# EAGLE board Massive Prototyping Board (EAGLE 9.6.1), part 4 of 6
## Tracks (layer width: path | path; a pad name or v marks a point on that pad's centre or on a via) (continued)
N$1187  (via drill 0.94) (continued)
  Bottom 2.032: v201.93,172.72 v204.47,172.72 v207.01,172.72 v209.55,172.72 v212.09,172.72
N$1188  (via drill 0.94)
  Bottom 2.032: v201.93,175.26 v204.47,175.26 v207.01,175.26 v209.55,175.26 v212.09,175.26
N$1189  (via drill 0.94)
  Bottom 2.032: v201.93,177.8 v204.47,177.8 v207.01,177.8 v209.55,177.8 v212.09,177.8
N$1190  (via drill 0.94)
  Bottom 2.032: v201.93,180.34 v204.47,180.34 v207.01,180.34 v209.55,180.34 v212.09,180.34
N$1191  (via drill 0.94)
  Bottom 2.032: v201.93,182.88 v204.47,182.88 v207.01,182.88 v209.55,182.88 v212.09,182.88
N$1192  (via drill 0.94)
  Bottom 2.032: v201.93,185.42 v204.47,185.42 v207.01,185.42 v209.55,185.42 v212.09,185.42
N$1193  (via drill 0.94)
  Bottom 2.032: v201.93,187.96 v204.47,187.96 v207.01,187.96 v209.55,187.96 v212.09,187.96
N$1194  (via drill 0.94)
  Bottom 2.032: v201.93,190.5 v204.47,190.5 v207.01,190.5 v209.55,190.5 v212.09,190.5
N$1195  (via drill 0.94)
  Bottom 2.032: v201.93,193.04 v204.47,193.04 v207.01,193.04 v209.55,193.04 v212.09,193.04
N$1196  (via drill 0.94)
  Bottom 2.032: v201.93,195.58 v204.47,195.58 v207.01,195.58 v209.55,195.58 v212.09,195.58
N$1197  (via drill 0.94)
  Bottom 2.032: v201.93,198.12 v204.47,198.12 v207.01,198.12 v209.55,198.12 v212.09,198.12
N$1198  (via drill 0.94)
  Bottom 2.032: v201.93,200.66 v204.47,200.66 v207.01,200.66 v209.55,200.66 v212.09,200.66
N$1199  (via drill 0.94)
  Bottom 2.032: v201.93,203.2 v204.47,203.2 v207.01,203.2 v209.55,203.2 v212.09,203.2
N$1200  (via drill 0.94)
  Bottom 2.032: v201.93,205.74 v204.47,205.74 v207.01,205.74 v209.55,205.74 v212.09,205.74
N$1201  (via drill 0.94)
  Bottom 2.032: v201.93,208.28 v204.47,208.28 v207.01,208.28 v209.55,208.28 v212.09,208.28
N$1202  (via drill 0.94)
  Bottom 2.032: v201.93,210.82 v204.47,210.82 v207.01,210.82 v209.55,210.82 v212.09,210.82
N$1203  (via drill 0.94)
  Bottom 2.032: v201.93,213.36 v204.47,213.36 v207.01,213.36 v209.55,213.36 v212.09,213.36
N$1204  (via drill 0.94)
  Bottom 2.032: v201.93,215.9 v204.47,215.9 v207.01,215.9 v209.55,215.9 v212.09,215.9
N$1205  (via drill 0.94)
  Bottom 2.032: v201.93,218.44 v204.47,218.44 v207.01,218.44 v209.55,218.44 v212.09,218.44
N$1206  (via drill 0.94)
  Bottom 2.032: v201.93,220.98 v204.47,220.98 v207.01,220.98 v209.55,220.98 v212.09,220.98
N$1207  (via drill 0.94)
  Bottom 2.032: v201.93,223.52 v204.47,223.52 v207.01,223.52 v209.55,223.52 v212.09,223.52
N$1208  (via drill 0.94)
  Bottom 2.032: v201.93,226.06 v204.47,226.06 v207.01,226.06 v209.55,226.06 v212.09,226.06
N$1209  (via drill 0.94)
  Bottom 2.032: v201.93,228.6 v204.47,228.6 v207.01,228.6 v209.55,228.6 v212.09,228.6
N$1210  (via drill 0.94)
  Bottom 2.032: v201.93,231.14 v204.47,231.14 v207.01,231.14 v209.55,231.14 v212.09,231.14
N$1211  (via drill 0.94)
  Bottom 2.032: v201.93,233.68 v204.47,233.68 v207.01,233.68 v209.55,233.68 v212.09,233.68
N$1212  (via drill 0.94)
  Bottom 2.032: v201.93,236.22 v204.47,236.22 v207.01,236.22 v209.55,236.22 v212.09,236.22
N$1213  (via drill 0.94)
  Bottom 2.032: v201.93,238.76 v204.47,238.76 v207.01,238.76 v209.55,238.76 v212.09,238.76
N$1214  (via drill 0.94)
  Bottom 2.032: v201.93,241.3 v204.47,241.3 v207.01,241.3 v209.55,241.3 v212.09,241.3
N$1215  (via drill 0.94)
  Bottom 2.032: v201.93,243.84 v204.47,243.84 v207.01,243.84 v209.55,243.84 v212.09,243.84
N$1216  (via drill 0.94)
  Bottom 2.032: v201.93,246.38 v204.47,246.38 v207.01,246.38 v209.55,246.38 v212.09,246.38
N$1217  (via drill 0.94)
  Bottom 2.032: v201.93,248.92 v204.47,248.92 v207.01,248.92 v209.55,248.92 v212.09,248.92
N$1218  (via drill 0.94)
  Bottom 2.032: v201.93,251.46 v204.47,251.46 v207.01,251.46 v209.55,251.46 v212.09,251.46
N$1219  (via drill 0.94)
  Bottom 2.032: v201.93,254 v204.47,254 v207.01,254 v209.55,254 v212.09,254
N$1220  (via drill 0.94)
  Bottom 2.032: v201.93,256.54 v204.47,256.54 v207.01,256.54 v209.55,256.54 v212.09,256.54
N$1221  (via drill 0.94)
  Bottom 2.032: v201.93,259.08 v204.47,259.08 v207.01,259.08 v209.55,259.08 v212.09,259.08
N$1222  (via drill 0.94)
  Bottom 2.032: v201.93,261.62 v204.47,261.62 v207.01,261.62 v209.55,261.62 v212.09,261.62
N$1223  (via drill 0.94)
  Bottom 2.032: v201.93,264.16 v204.47,264.16 v207.01,264.16 v209.55,264.16 v212.09,264.16
N$1224  (via drill 0.94)
  Bottom 2.032: v201.93,266.7 v204.47,266.7 v207.01,266.7 v209.55,266.7 v212.09,266.7
N$1225  (via drill 0.94)
  Bottom 2.032: v201.93,269.24 v204.47,269.24 v207.01,269.24 v209.55,269.24 v212.09,269.24
N$1226  (via drill 0.94)
  Bottom 2.032: v201.93,271.78 v204.47,271.78 v207.01,271.78 v209.55,271.78 v212.09,271.78
N$1227  (via drill 0.94)
  Bottom 2.032: v201.93,274.32 v204.47,274.32 v207.01,274.32 v209.55,274.32 v212.09,274.32
N$1228  (via drill 0.94)
  Bottom 2.032: v201.93,276.86 v204.47,276.86 v207.01,276.86 v209.55,276.86 v212.09,276.86
N$1229  (via drill 0.94)
  Bottom 2.032: v219.71,12.7 v222.25,12.7 v224.79,12.7 v227.33,12.7 v229.87,12.7
N$1230  (via drill 0.94)
  Bottom 2.032: v219.71,15.24 v222.25,15.24 v224.79,15.24 v227.33,15.24 v229.87,15.24
N$1231  (via drill 0.94)
  Bottom 2.032: v219.71,17.78 v222.25,17.78 v224.79,17.78 v227.33,17.78 v229.87,17.78
N$1232  (via drill 0.94)
  Bottom 2.032: v219.71,20.32 v222.25,20.32 v224.79,20.32 v227.33,20.32 v229.87,20.32
N$1233  (via drill 0.94)
  Bottom 2.032: v219.71,22.86 v222.25,22.86 v224.79,22.86 v227.33,22.86 v229.87,22.86
N$1234  (via drill 0.94)
  Bottom 2.032: v219.71,25.4 v222.25,25.4 v224.79,25.4 v227.33,25.4 v229.87,25.4
N$1235  (via drill 0.94)
  Bottom 2.032: v219.71,27.94 v222.25,27.94 v224.79,27.94 v227.33,27.94 v229.87,27.94
N$1236  (via drill 0.94)
  Bottom 2.032: v219.71,30.48 v222.25,30.48 v224.79,30.48 v227.33,30.48 v229.87,30.48
N$1237  (via drill 0.94)
  Bottom 2.032: v219.71,33.02 v222.25,33.02 v224.79,33.02 v227.33,33.02 v229.87,33.02
N$1238  (via drill 0.94)
  Bottom 2.032: v219.71,35.56 v222.25,35.56 v224.79,35.56 v227.33,35.56 v229.87,35.56
N$1239  (via drill 0.94)
  Bottom 2.032: v219.71,38.1 v222.25,38.1 v224.79,38.1 v227.33,38.1 v229.87,38.1
N$1240  (via drill 0.94)
  Bottom 2.032: v219.71,40.64 v222.25,40.64 v224.79,40.64 v227.33,40.64 v229.87,40.64
N$1241  (via drill 0.94)
  Bottom 2.032: v219.71,43.18 v222.25,43.18 v224.79,43.18 v227.33,43.18 v229.87,43.18
N$1242  (via drill 0.94)
  Bottom 2.032: v219.71,45.72 v222.25,45.72 v224.79,45.72 v227.33,45.72 v229.87,45.72
N$1243  (via drill 0.94)
  Bottom 2.032: v219.71,48.26 v222.25,48.26 v224.79,48.26 v227.33,48.26 v229.87,48.26
N$1244  (via drill 0.94)
  Bottom 2.032: v219.71,50.8 v222.25,50.8 v224.79,50.8 v227.33,50.8 v229.87,50.8
N$1245  (via drill 0.94)
  Bottom 2.032: v219.71,53.34 v222.25,53.34 v224.79,53.34 v227.33,53.34 v229.87,53.34
N$1246  (via drill 0.94)
  Bottom 2.032: v219.71,55.88 v222.25,55.88 v224.79,55.88 v227.33,55.88 v229.87,55.88
N$1247  (via drill 0.94)
  Bottom 2.032: v219.71,58.42 v222.25,58.42 v224.79,58.42 v227.33,58.42 v229.87,58.42
N$1248  (via drill 0.94)
  Bottom 2.032: v219.71,60.96 v222.25,60.96 v224.79,60.96 v227.33,60.96 v229.87,60.96
N$1249  (via drill 0.94)
  Bottom 2.032: v219.71,63.5 v222.25,63.5 v224.79,63.5 v227.33,63.5 v229.87,63.5
N$1250  (via drill 0.94)
  Bottom 2.032: v219.71,66.04 v222.25,66.04 v224.79,66.04 v227.33,66.04 v229.87,66.04
N$1251  (via drill 0.94)
  Bottom 2.032: v219.71,68.58 v222.25,68.58 v224.79,68.58 v227.33,68.58 v229.87,68.58
N$1252  (via drill 0.94)
  Bottom 2.032: v219.71,71.12 v222.25,71.12 v224.79,71.12 v227.33,71.12 v229.87,71.12
N$1253  (via drill 0.94)
  Bottom 2.032: v219.71,73.66 v222.25,73.66 v224.79,73.66 v227.33,73.66 v229.87,73.66
N$1254  (via drill 0.94)
  Bottom 2.032: v219.71,76.2 v222.25,76.2 v224.79,76.2 v227.33,76.2 v229.87,76.2
N$1255  (via drill 0.94)
  Bottom 2.032: v219.71,78.74 v222.25,78.74 v224.79,78.74 v227.33,78.74 v229.87,78.74
N$1256  (via drill 0.94)
  Bottom 2.032: v219.71,81.28 v222.25,81.28 v224.79,81.28 v227.33,81.28 v229.87,81.28
N$1257  (via drill 0.94)
  Bottom 2.032: v219.71,83.82 v222.25,83.82 v224.79,83.82 v227.33,83.82 v229.87,83.82
N$1258  (via drill 0.94)
  Bottom 2.032: v219.71,86.36 v222.25,86.36 v224.79,86.36 v227.33,86.36 v229.87,86.36
N$1259  (via drill 0.94)
  Bottom 2.032: v219.71,88.9 v222.25,88.9 v224.79,88.9 v227.33,88.9 v229.87,88.9
N$1260  (via drill 0.94)
  Bottom 2.032: v219.71,91.44 v222.25,91.44 v224.79,91.44 v227.33,91.44 v229.87,91.44
N$1261  (via drill 0.94)
  Bottom 2.032: v219.71,93.98 v222.25,93.98 v224.79,93.98 v227.33,93.98 v229.87,93.98
N$1262  (via drill 0.94)
  Bottom 2.032: v219.71,96.52 v222.25,96.52 v224.79,96.52 v227.33,96.52 v229.87,96.52
N$1263  (via drill 0.94)
  Bottom 2.032: v219.71,99.06 v222.25,99.06 v224.79,99.06 v227.33,99.06 v229.87,99.06
N$1264  (via drill 0.94)
  Bottom 2.032: v219.71,101.6 v222.25,101.6 v224.79,101.6 v227.33,101.6 v229.87,101.6
N$1265  (via drill 0.94)
  Bottom 2.032: v219.71,104.14 v222.25,104.14 v224.79,104.14 v227.33,104.14 v229.87,104.14
N$1266  (via drill 0.94)
  Bottom 2.032: v219.71,106.68 v222.25,106.68 v224.79,106.68 v227.33,106.68 v229.87,106.68
N$1267  (via drill 0.94)
  Bottom 2.032: v219.71,109.22 v222.25,109.22 v224.79,109.22 v227.33,109.22 v229.87,109.22
N$1268  (via drill 0.94)
  Bottom 2.032: v219.71,111.76 v222.25,111.76 v224.79,111.76 v227.33,111.76 v229.87,111.76
N$1269  (via drill 0.94)
  Bottom 2.032: v219.71,114.3 v222.25,114.3 v224.79,114.3 v227.33,114.3 v229.87,114.3
N$1270  (via drill 0.94)
  Bottom 2.032: v219.71,116.84 v222.25,116.84 v224.79,116.84 v227.33,116.84 v229.87,116.84
N$1271  (via drill 0.94)
  Bottom 2.032: v219.71,119.38 v222.25,119.38 v224.79,119.38 v227.33,119.38 v229.87,119.38
N$1272  (via drill 0.94)
  Bottom 2.032: v219.71,121.92 v222.25,121.92 v224.79,121.92 v227.33,121.92 v229.87,121.92
N$1273  (via drill 0.94)
  Bottom 2.032: v219.71,124.46 v222.25,124.46 v224.79,124.46 v227.33,124.46 v229.87,124.46
N$1274  (via drill 0.94)
  Bottom 2.032: v219.71,127 v222.25,127 v224.79,127 v227.33,127 v229.87,127
N$1275  (via drill 0.94)
  Bottom 2.032: v219.71,129.54 v222.25,129.54 v224.79,129.54 v227.33,129.54 v229.87,129.54
N$1276  (via drill 0.94)
  Bottom 2.032: v219.71,132.08 v222.25,132.08 v224.79,132.08 v227.33,132.08 v229.87,132.08
N$1277  (via drill 0.94)
  Bottom 2.032: v219.71,134.62 v222.25,134.62 v224.79,134.62 v227.33,134.62 v229.87,134.62
N$1278  (via drill 0.94)
  Bottom 2.032: v219.71,137.16 v222.25,137.16 v224.79,137.16 v227.33,137.16 v229.87,137.16
N$1279  (via drill 0.94)
  Bottom 2.032: v219.71,139.7 v222.25,139.7 v224.79,139.7 v227.33,139.7 v229.87,139.7
N$1280  (via drill 0.94)
  Bottom 2.032: v219.71,142.24 v222.25,142.24 v224.79,142.24 v227.33,142.24 v229.87,142.24
N$1281  (via drill 0.94)
  Bottom 2.032: v219.71,144.78 v222.25,144.78 v224.79,144.78 v227.33,144.78 v229.87,144.78
N$1282  (via drill 0.94)
  Bottom 2.032: v219.71,147.32 v222.25,147.32 v224.79,147.32 v227.33,147.32 v229.87,147.32
N$1283  (via drill 0.94)
  Bottom 2.032: v219.71,149.86 v222.25,149.86 v224.79,149.86 v227.33,149.86 v229.87,149.86
N$1284  (via drill 0.94)
  Bottom 2.032: v219.71,152.4 v222.25,152.4 v224.79,152.4 v227.33,152.4 v229.87,152.4
N$1285  (via drill 0.94)
  Bottom 2.032: v219.71,154.94 v222.25,154.94 v224.79,154.94 v227.33,154.94 v229.87,154.94
N$1286  (via drill 0.94)
  Bottom 2.032: v219.71,157.48 v222.25,157.48 v224.79,157.48 v227.33,157.48 v229.87,157.48
N$1287  (via drill 0.94)
  Bottom 2.032: v219.71,160.02 v222.25,160.02 v224.79,160.02 v227.33,160.02 v229.87,160.02
N$1288  (via drill 0.94)
  Bottom 2.032: v219.71,162.56 v222.25,162.56 v224.79,162.56 v227.33,162.56 v229.87,162.56
N$1289  (via drill 0.94)
  Bottom 2.032: v219.71,165.1 v222.25,165.1 v224.79,165.1 v227.33,165.1 v229.87,165.1
N$1290  (via drill 0.94)
  Bottom 2.032: v219.71,167.64 v222.25,167.64 v224.79,167.64 v227.33,167.64 v229.87,167.64
N$1291  (via drill 0.94)
  Bottom 2.032: v219.71,170.18 v222.25,170.18 v224.79,170.18 v227.33,170.18 v229.87,170.18
N$1292  (via drill 0.94)
  Bottom 2.032: v219.71,172.72 v222.25,172.72 v224.79,172.72 v227.33,172.72 v229.87,172.72
N$1293  (via drill 0.94)
  Bottom 2.032: v219.71,175.26 v222.25,175.26 v224.79,175.26 v227.33,175.26 v229.87,175.26
N$1294  (via drill 0.94)
  Bottom 2.032: v219.71,177.8 v222.25,177.8 v224.79,177.8 v227.33,177.8 v229.87,177.8
N$1295  (via drill 0.94)
  Bottom 2.032: v219.71,180.34 v222.25,180.34 v224.79,180.34 v227.33,180.34 v229.87,180.34
N$1296  (via drill 0.94)
  Bottom 2.032: v219.71,182.88 v222.25,182.88 v224.79,182.88 v227.33,182.88 v229.87,182.88
N$1297  (via drill 0.94)
  Bottom 2.032: v219.71,185.42 v222.25,185.42 v224.79,185.42 v227.33,185.42 v229.87,185.42
N$1298  (via drill 0.94)
  Bottom 2.032: v219.71,187.96 v222.25,187.96 v224.79,187.96 v227.33,187.96 v229.87,187.96
N$1299  (via drill 0.94)
  Bottom 2.032: v219.71,190.5 v222.25,190.5 v224.79,190.5 v227.33,190.5 v229.87,190.5
N$1300  (via drill 0.94)
  Bottom 2.032: v219.71,193.04 v222.25,193.04 v224.79,193.04 v227.33,193.04 v229.87,193.04
N$1301  (via drill 0.94)
  Bottom 2.032: v219.71,195.58 v222.25,195.58 v224.79,195.58 v227.33,195.58 v229.87,195.58
N$1302  (via drill 0.94)
  Bottom 2.032: v219.71,198.12 v222.25,198.12 v224.79,198.12 v227.33,198.12 v229.87,198.12
N$1303  (via drill 0.94)
  Bottom 2.032: v219.71,200.66 v222.25,200.66 v224.79,200.66 v227.33,200.66 v229.87,200.66
N$1304  (via drill 0.94)
  Bottom 2.032: v219.71,203.2 v222.25,203.2 v224.79,203.2 v227.33,203.2 v229.87,203.2
N$1305  (via drill 0.94)
  Bottom 2.032: v219.71,205.74 v222.25,205.74 v224.79,205.74 v227.33,205.74 v229.87,205.74
N$1306  (via drill 0.94)
  Bottom 2.032: v219.71,208.28 v222.25,208.28 v224.79,208.28 v227.33,208.28 v229.87,208.28
N$1307  (via drill 0.94)
  Bottom 2.032: v219.71,210.82 v222.25,210.82 v224.79,210.82 v227.33,210.82 v229.87,210.82
N$1308  (via drill 0.94)
  Bottom 2.032: v219.71,213.36 v222.25,213.36 v224.79,213.36 v227.33,213.36 v229.87,213.36
N$1309  (via drill 0.94)
  Bottom 2.032: v219.71,215.9 v222.25,215.9 v224.79,215.9 v227.33,215.9 v229.87,215.9
N$1310  (via drill 0.94)
  Bottom 2.032: v219.71,218.44 v222.25,218.44 v224.79,218.44 v227.33,218.44 v229.87,218.44
N$1311  (via drill 0.94)
  Bottom 2.032: v219.71,220.98 v222.25,220.98 v224.79,220.98 v227.33,220.98 v229.87,220.98
N$1312  (via drill 0.94)
  Bottom 2.032: v219.71,223.52 v222.25,223.52 v224.79,223.52 v227.33,223.52 v229.87,223.52
N$1313  (via drill 0.94)
  Bottom 2.032: v219.71,226.06 v222.25,226.06 v224.79,226.06 v227.33,226.06 v229.87,226.06
N$1314  (via drill 0.94)
  Bottom 2.032: v219.71,228.6 v222.25,228.6 v224.79,228.6 v227.33,228.6 v229.87,228.6
N$1315  (via drill 0.94)
  Bottom 2.032: v219.71,231.14 v222.25,231.14 v224.79,231.14 v227.33,231.14 v229.87,231.14
N$1316  (via drill 0.94)
  Bottom 2.032: v219.71,233.68 v222.25,233.68 v224.79,233.68 v227.33,233.68 v229.87,233.68
N$1317  (via drill 0.94)
  Bottom 2.032: v219.71,236.22 v222.25,236.22 v224.79,236.22 v227.33,236.22 v229.87,236.22
N$1318  (via drill 0.94)
  Bottom 2.032: v219.71,238.76 v222.25,238.76 v224.79,238.76 v227.33,238.76 v229.87,238.76
N$1319  (via drill 0.94)
  Bottom 2.032: v219.71,241.3 v222.25,241.3 v224.79,241.3 v227.33,241.3 v229.87,241.3
N$1320  (via drill 0.94)
  Bottom 2.032: v219.71,243.84 v222.25,243.84 v224.79,243.84 v227.33,243.84 v229.87,243.84
N$1321  (via drill 0.94)
  Bottom 2.032: v219.71,246.38 v222.25,246.38 v224.79,246.38 v227.33,246.38 v229.87,246.38
N$1322  (via drill 0.94)
  Bottom 2.032: v219.71,248.92 v222.25,248.92 v224.79,248.92 v227.33,248.92 v229.87,248.92
N$1323  (via drill 0.94)
  Bottom 2.032: v219.71,251.46 v222.25,251.46 v224.79,251.46 v227.33,251.46 v229.87,251.46
N$1324  (via drill 0.94)
  Bottom 2.032: v219.71,254 v222.25,254 v224.79,254 v227.33,254 v229.87,254
N$1325  (via drill 0.94)
  Bottom 2.032: v219.71,256.54 v222.25,256.54 v224.79,256.54 v227.33,256.54 v229.87,256.54
N$1326  (via drill 0.94)
  Bottom 2.032: v219.71,259.08 v222.25,259.08 v224.79,259.08 v227.33,259.08 v229.87,259.08
N$1327  (via drill 0.94)
  Bottom 2.032: v219.71,261.62 v222.25,261.62 v224.79,261.62 v227.33,261.62 v229.87,261.62
N$1328  (via drill 0.94)
  Bottom 2.032: v219.71,264.16 v222.25,264.16 v224.79,264.16 v227.33,264.16 v229.87,264.16
N$1329  (via drill 0.94)
  Bottom 2.032: v219.71,266.7 v222.25,266.7 v224.79,266.7 v227.33,266.7 v229.87,266.7
N$1330  (via drill 0.94)
  Bottom 2.032: v219.71,269.24 v222.25,269.24 v224.79,269.24 v227.33,269.24 v229.87,269.24
N$1331  (via drill 0.94)
  Bottom 2.032: v219.71,271.78 v222.25,271.78 v224.79,271.78 v227.33,271.78 v229.87,271.78
N$1332  (via drill 0.94)
  Bottom 2.032: v219.71,274.32 v222.25,274.32 v224.79,274.32 v227.33,274.32 v229.87,274.32
N$1333  (via drill 0.94)
  Bottom 2.032: v219.71,276.86 v222.25,276.86 v224.79,276.86 v227.33,276.86 v229.87,276.86
N$1334  (via drill 0.94)
  Bottom 2.032: v232.41,12.7 v234.95,12.7 v237.49,12.7 v240.03,12.7 v242.57,12.7
N$1335  (via drill 0.94)
  Bottom 2.032: v232.41,15.24 v234.95,15.24 v237.49,15.24 v240.03,15.24 v242.57,15.24
N$1336  (via drill 0.94)
  Bottom 2.032: v232.41,17.78 v234.95,17.78 v237.49,17.78 v240.03,17.78 v242.57,17.78
N$1337  (via drill 0.94)
  Bottom 2.032: v232.41,20.32 v234.95,20.32 v237.49,20.32 v240.03,20.32 v242.57,20.32
N$1338  (via drill 0.94)
  Bottom 2.032: v232.41,22.86 v234.95,22.86 v237.49,22.86 v240.03,22.86 v242.57,22.86
N$1339  (via drill 0.94)
  Bottom 2.032: v232.41,25.4 v234.95,25.4 v237.49,25.4 v240.03,25.4 v242.57,25.4
N$1340  (via drill 0.94)
  Bottom 2.032: v232.41,27.94 v234.95,27.94 v237.49,27.94 v240.03,27.94 v242.57,27.94
N$1341  (via drill 0.94)
  Bottom 2.032: v232.41,30.48 v234.95,30.48 v237.49,30.48 v240.03,30.48 v242.57,30.48
N$1342  (via drill 0.94)
  Bottom 2.032: v232.41,33.02 v234.95,33.02 v237.49,33.02 v240.03,33.02 v242.57,33.02
N$1343  (via drill 0.94)
  Bottom 2.032: v232.41,35.56 v234.95,35.56 v237.49,35.56 v240.03,35.56 v242.57,35.56
N$1344  (via drill 0.94)
  Bottom 2.032: v232.41,38.1 v234.95,38.1 v237.49,38.1 v240.03,38.1 v242.57,38.1
N$1345  (via drill 0.94)
  Bottom 2.032: v232.41,40.64 v234.95,40.64 v237.49,40.64 v240.03,40.64 v242.57,40.64
N$1346  (via drill 0.94)
  Bottom 2.032: v232.41,43.18 v234.95,43.18 v237.49,43.18 v240.03,43.18 v242.57,43.18
N$1347  (via drill 0.94)
  Bottom 2.032: v232.41,45.72 v234.95,45.72 v237.49,45.72 v240.03,45.72 v242.57,45.72
N$1348  (via drill 0.94)
  Bottom 2.032: v232.41,48.26 v234.95,48.26 v237.49,48.26 v240.03,48.26 v242.57,48.26
N$1349  (via drill 0.94)
  Bottom 2.032: v232.41,50.8 v234.95,50.8 v237.49,50.8 v240.03,50.8 v242.57,50.8
N$1350  (via drill 0.94)
  Bottom 2.032: v232.41,53.34 v234.95,53.34 v237.49,53.34 v240.03,53.34 v242.57,53.34
N$1351  (via drill 0.94)
  Bottom 2.032: v232.41,55.88 v234.95,55.88 v237.49,55.88 v240.03,55.88 v242.57,55.88
N$1352  (via drill 0.94)
  Bottom 2.032: v232.41,58.42 v234.95,58.42 v237.49,58.42 v240.03,58.42 v242.57,58.42
N$1353  (via drill 0.94)
  Bottom 2.032: v232.41,60.96 v234.95,60.96 v237.49,60.96 v240.03,60.96 v242.57,60.96
N$1354  (via drill 0.94)
  Bottom 2.032: v232.41,63.5 v234.95,63.5 v237.49,63.5 v240.03,63.5 v242.57,63.5
N$1355  (via drill 0.94)
  Bottom 2.032: v232.41,66.04 v234.95,66.04 v237.49,66.04 v240.03,66.04 v242.57,66.04
N$1356  (via drill 0.94)
  Bottom 2.032: v232.41,68.58 v234.95,68.58 v237.49,68.58 v240.03,68.58 v242.57,68.58
N$1357  (via drill 0.94)
  Bottom 2.032: v232.41,71.12 v234.95,71.12 v237.49,71.12 v240.03,71.12 v242.57,71.12
N$1358  (via drill 0.94)
  Bottom 2.032: v232.41,73.66 v234.95,73.66 v237.49,73.66 v240.03,73.66 v242.57,73.66
N$1359  (via drill 0.94)
  Bottom 2.032: v232.41,76.2 v234.95,76.2 v237.49,76.2 v240.03,76.2 v242.57,76.2
N$1360  (via drill 0.94)
  Bottom 2.032: v232.41,78.74 v234.95,78.74 v237.49,78.74 v240.03,78.74 v242.57,78.74
N$1361  (via drill 0.94)
  Bottom 2.032: v232.41,81.28 v234.95,81.28 v237.49,81.28 v240.03,81.28 v242.57,81.28
N$1362  (via drill 0.94)
  Bottom 2.032: v232.41,83.82 v234.95,83.82 v237.49,83.82 v240.03,83.82 v242.57,83.82
N$1363  (via drill 0.94)
  Bottom 2.032: v232.41,86.36 v234.95,86.36 v237.49,86.36 v240.03,86.36 v242.57,86.36
N$1364  (via drill 0.94)
  Bottom 2.032: v232.41,88.9 v234.95,88.9 v237.49,88.9 v240.03,88.9 v242.57,88.9
N$1365  (via drill 0.94)
  Bottom 2.032: v232.41,91.44 v234.95,91.44 v237.49,91.44 v240.03,91.44 v242.57,91.44
N$1366  (via drill 0.94)
  Bottom 2.032: v232.41,93.98 v234.95,93.98 v237.49,93.98 v240.03,93.98 v242.57,93.98
N$1367  (via drill 0.94)
  Bottom 2.032: v232.41,96.52 v234.95,96.52 v237.49,96.52 v240.03,96.52 v242.57,96.52
N$1368  (via drill 0.94)
  Bottom 2.032: v232.41,99.06 v234.95,99.06 v237.49,99.06 v240.03,99.06 v242.57,99.06
N$1369  (via drill 0.94)
  Bottom 2.032: v232.41,101.6 v234.95,101.6 v237.49,101.6 v240.03,101.6 v242.57,101.6
N$1370  (via drill 0.94)
  Bottom 2.032: v232.41,104.14 v234.95,104.14 v237.49,104.14 v240.03,104.14 v242.57,104.14
N$1371  (via drill 0.94)
  Bottom 2.032: v232.41,106.68 v234.95,106.68 v237.49,106.68 v240.03,106.68 v242.57,106.68
N$1372  (via drill 0.94)
  Bottom 2.032: v232.41,109.22 v234.95,109.22 v237.49,109.22 v240.03,109.22 v242.57,109.22
N$1373  (via drill 0.94)
  Bottom 2.032: v232.41,111.76 v234.95,111.76 v237.49,111.76 v240.03,111.76 v242.57,111.76
N$1374  (via drill 0.94)
  Bottom 2.032: v232.41,114.3 v234.95,114.3 v237.49,114.3 v240.03,114.3 v242.57,114.3
N$1375  (via drill 0.94)
  Bottom 2.032: v232.41,116.84 v234.95,116.84 v237.49,116.84 v240.03,116.84 v242.57,116.84
N$1376  (via drill 0.94)
  Bottom 2.032: v232.41,119.38 v234.95,119.38 v237.49,119.38 v240.03,119.38 v242.57,119.38
N$1377  (via drill 0.94)
  Bottom 2.032: v232.41,121.92 v234.95,121.92 v237.49,121.92 v240.03,121.92 v242.57,121.92
N$1378  (via drill 0.94)
  Bottom 2.032: v232.41,124.46 v234.95,124.46 v237.49,124.46 v240.03,124.46 v242.57,124.46
N$1379  (via drill 0.94)
  Bottom 2.032: v232.41,127 v234.95,127 v237.49,127 v240.03,127 v242.57,127
N$1380  (via drill 0.94)
  Bottom 2.032: v232.41,129.54 v234.95,129.54 v237.49,129.54 v240.03,129.54 v242.57,129.54
N$1381  (via drill 0.94)
  Bottom 2.032: v232.41,132.08 v234.95,132.08 v237.49,132.08 v240.03,132.08 v242.57,132.08
N$1382  (via drill 0.94)
  Bottom 2.032: v232.41,134.62 v234.95,134.62 v237.49,134.62 v240.03,134.62 v242.57,134.62
N$1383  (via drill 0.94)
  Bottom 2.032: v232.41,137.16 v234.95,137.16 v237.49,137.16 v240.03,137.16 v242.57,137.16
N$1384  (via drill 0.94)
  Bottom 2.032: v232.41,139.7 v234.95,139.7 v237.49,139.7 v240.03,139.7 v242.57,139.7
N$1385  (via drill 0.94)
  Bottom 2.032: v232.41,142.24 v234.95,142.24 v237.49,142.24 v240.03,142.24 v242.57,142.24
N$1386  (via drill 0.94)
  Bottom 2.032: v232.41,144.78 v234.95,144.78 v237.49,144.78 v240.03,144.78 v242.57,144.78
N$1387  (via drill 0.94)
  Bottom 2.032: v232.41,147.32 v234.95,147.32 v237.49,147.32 v240.03,147.32 v242.57,147.32
N$1388  (via drill 0.94)
  Bottom 2.032: v232.41,149.86 v234.95,149.86 v237.49,149.86 v240.03,149.86 v242.57,149.86
N$1389  (via drill 0.94)
  Bottom 2.032: v232.41,152.4 v234.95,152.4 v237.49,152.4 v240.03,152.4 v242.57,152.4
N$1390  (via drill 0.94)
  Bottom 2.032: v232.41,154.94 v234.95,154.94 v237.49,154.94 v240.03,154.94 v242.57,154.94
N$1391  (via drill 0.94)
  Bottom 2.032: v232.41,157.48 v234.95,157.48 v237.49,157.48 v240.03,157.48 v242.57,157.48
N$1392  (via drill 0.94)
  Bottom 2.032: v232.41,160.02 v234.95,160.02 v237.49,160.02 v240.03,160.02 v242.57,160.02
N$1393  (via drill 0.94)
  Bottom 2.032: v232.41,162.56 v234.95,162.56 v237.49,162.56 v240.03,162.56 v242.57,162.56
N$1394  (via drill 0.94)
  Bottom 2.032: v232.41,165.1 v234.95,165.1 v237.49,165.1 v240.03,165.1 v242.57,165.1
N$1395  (via drill 0.94)
  Bottom 2.032: v232.41,167.64 v234.95,167.64 v237.49,167.64 v240.03,167.64 v242.57,167.64
N$1396  (via drill 0.94)
  Bottom 2.032: v232.41,170.18 v234.95,170.18 v237.49,170.18 v240.03,170.18 v242.57,170.18
N$1397  (via drill 0.94)
  Bottom 2.032: v232.41,172.72 v234.95,172.72 v237.49,172.72 v240.03,172.72 v242.57,172.72
N$1398  (via drill 0.94)
  Bottom 2.032: v232.41,175.26 v234.95,175.26 v237.49,175.26 v240.03,175.26 v242.57,175.26
N$1399  (via drill 0.94)
  Bottom 2.032: v232.41,177.8 v234.95,177.8 v237.49,177.8 v240.03,177.8 v242.57,177.8
N$1400  (via drill 0.94)
  Bottom 2.032: v232.41,180.34 v234.95,180.34 v237.49,180.34 v240.03,180.34 v242.57,180.34
N$1401  (via drill 0.94)
  Bottom 2.032: v232.41,182.88 v234.95,182.88 v237.49,182.88 v240.03,182.88 v242.57,182.88
N$1402  (via drill 0.94)
  Bottom 2.032: v232.41,185.42 v234.95,185.42 v237.49,185.42 v240.03,185.42 v242.57,185.42
N$1403  (via drill 0.94)
  Bottom 2.032: v232.41,187.96 v234.95,187.96 v237.49,187.96 v240.03,187.96 v242.57,187.96
N$1404  (via drill 0.94)
  Bottom 2.032: v232.41,190.5 v234.95,190.5 v237.49,190.5 v240.03,190.5 v242.57,190.5
N$1405  (via drill 0.94)
  Bottom 2.032: v232.41,193.04 v234.95,193.04 v237.49,193.04 v240.03,193.04 v242.57,193.04
N$1406  (via drill 0.94)
  Bottom 2.032: v232.41,195.58 v234.95,195.58 v237.49,195.58 v240.03,195.58 v242.57,195.58
N$1407  (via drill 0.94)
  Bottom 2.032: v232.41,198.12 v234.95,198.12 v237.49,198.12 v240.03,198.12 v242.57,198.12
N$1408  (via drill 0.94)
  Bottom 2.032: v232.41,200.66 v234.95,200.66 v237.49,200.66 v240.03,200.66 v242.57,200.66
N$1409  (via drill 0.94)
  Bottom 2.032: v232.41,203.2 v234.95,203.2 v237.49,203.2 v240.03,203.2 v242.57,203.2
N$1410  (via drill 0.94)
  Bottom 2.032: v232.41,205.74 v234.95,205.74 v237.49,205.74 v240.03,205.74 v242.57,205.74
N$1411  (via drill 0.94)
  Bottom 2.032: v232.41,208.28 v234.95,208.28 v237.49,208.28 v240.03,208.28 v242.57,208.28
N$1412  (via drill 0.94)
  Bottom 2.032: v232.41,210.82 v234.95,210.82 v237.49,210.82 v240.03,210.82 v242.57,210.82
N$1413  (via drill 0.94)
  Bottom 2.032: v232.41,213.36 v234.95,213.36 v237.49,213.36 v240.03,213.36 v242.57,213.36
N$1414  (via drill 0.94)
  Bottom 2.032: v232.41,215.9 v234.95,215.9 v237.49,215.9 v240.03,215.9 v242.57,215.9
N$1415  (via drill 0.94)
  Bottom 2.032: v232.41,218.44 v234.95,218.44 v237.49,218.44 v240.03,218.44 v242.57,218.44
N$1416  (via drill 0.94)
  Bottom 2.032: v232.41,220.98 v234.95,220.98 v237.49,220.98 v240.03,220.98 v242.57,220.98
N$1417  (via drill 0.94)
  Bottom 2.032: v232.41,223.52 v234.95,223.52 v237.49,223.52 v240.03,223.52 v242.57,223.52
N$1418  (via drill 0.94)
  Bottom 2.032: v232.41,226.06 v234.95,226.06 v237.49,226.06 v240.03,226.06 v242.57,226.06
N$1419  (via drill 0.94)
  Bottom 2.032: v232.41,228.6 v234.95,228.6 v237.49,228.6 v240.03,228.6 v242.57,228.6
N$1420  (via drill 0.94)
  Bottom 2.032: v232.41,231.14 v234.95,231.14 v237.49,231.14 v240.03,231.14 v242.57,231.14
N$1421  (via drill 0.94)
  Bottom 2.032: v232.41,233.68 v234.95,233.68 v237.49,233.68 v240.03,233.68 v242.57,233.68
N$1422  (via drill 0.94)
  Bottom 2.032: v232.41,236.22 v234.95,236.22 v237.49,236.22 v240.03,236.22 v242.57,236.22
N$1423  (via drill 0.94)
  Bottom 2.032: v232.41,238.76 v234.95,238.76 v237.49,238.76 v240.03,238.76 v242.57,238.76
N$1424  (via drill 0.94)
  Bottom 2.032: v232.41,241.3 v234.95,241.3 v237.49,241.3 v240.03,241.3 v242.57,241.3
N$1425  (via drill 0.94)
  Bottom 2.032: v232.41,243.84 v234.95,243.84 v237.49,243.84 v240.03,243.84 v242.57,243.84
N$1426  (via drill 0.94)
  Bottom 2.032: v232.41,246.38 v234.95,246.38 v237.49,246.38 v240.03,246.38 v242.57,246.38
N$1427  (via drill 0.94)
  Bottom 2.032: v232.41,248.92 v234.95,248.92 v237.49,248.92 v240.03,248.92 v242.57,248.92
N$1428  (via drill 0.94)
  Bottom 2.032: v232.41,251.46 v234.95,251.46 v237.49,251.46 v240.03,251.46 v242.57,251.46
N$1429  (via drill 0.94)
  Bottom 2.032: v232.41,254 v234.95,254 v237.49,254 v240.03,254 v242.57,254
N$1430  (via drill 0.94)
  Bottom 2.032: v232.41,256.54 v234.95,256.54 v237.49,256.54 v240.03,256.54 v242.57,256.54
N$1431  (via drill 0.94)
  Bottom 2.032: v232.41,259.08 v234.95,259.08 v237.49,259.08 v240.03,259.08 v242.57,259.08
N$1432  (via drill 0.94)
  Bottom 2.032: v232.41,261.62 v234.95,261.62 v237.49,261.62 v240.03,261.62 v242.57,261.62
N$1433  (via drill 0.94)
  Bottom 2.032: v232.41,264.16 v234.95,264.16 v237.49,264.16 v240.03,264.16 v242.57,264.16
N$1434  (via drill 0.94)
  Bottom 2.032: v232.41,266.7 v234.95,266.7 v237.49,266.7 v240.03,266.7 v242.57,266.7
N$1435  (via drill 0.94)
  Bottom 2.032: v232.41,269.24 v234.95,269.24 v237.49,269.24 v240.03,269.24 v242.57,269.24
N$1436  (via drill 0.94)
  Bottom 2.032: v232.41,271.78 v234.95,271.78 v237.49,271.78 v240.03,271.78 v242.57,271.78
N$1437  (via drill 0.94)
  Bottom 2.032: v232.41,274.32 v234.95,274.32 v237.49,274.32 v240.03,274.32 v242.57,274.32
N$1438  (via drill 0.94)
  Bottom 2.032: v232.41,276.86 v234.95,276.86 v237.49,276.86 v240.03,276.86 v242.57,276.86
N$1439  (via drill 0.94)
  Bottom 2.032: v250.19,12.7 v252.73,12.7 v255.27,12.7 v257.81,12.7 v260.35,12.7
N$1440  (via drill 0.94)
  Bottom 2.032: v250.19,15.24 v252.73,15.24 v255.27,15.24 v257.81,15.24 v260.35,15.24
N$1441  (via drill 0.94)
  Bottom 2.032: v250.19,17.78 v252.73,17.78 v255.27,17.78 v257.81,17.78 v260.35,17.78
N$1442  (via drill 0.94)
  Bottom 2.032: v250.19,20.32 v252.73,20.32 v255.27,20.32 v257.81,20.32 v260.35,20.32
N$1443  (via drill 0.94)
  Bottom 2.032: v250.19,22.86 v252.73,22.86 v255.27,22.86 v257.81,22.86 v260.35,22.86
N$1444  (via drill 0.94)
  Bottom 2.032: v250.19,25.4 v252.73,25.4 v255.27,25.4 v257.81,25.4 v260.35,25.4
N$1445  (via drill 0.94)
  Bottom 2.032: v250.19,27.94 v252.73,27.94 v255.27,27.94 v257.81,27.94 v260.35,27.94
N$1446  (via drill 0.94)
  Bottom 2.032: v250.19,30.48 v252.73,30.48 v255.27,30.48 v257.81,30.48 v260.35,30.48
N$1447  (via drill 0.94)
  Bottom 2.032: v250.19,33.02 v252.73,33.02 v255.27,33.02 v257.81,33.02 v260.35,33.02
N$1448  (via drill 0.94)
  Bottom 2.032: v250.19,35.56 v252.73,35.56 v255.27,35.56 v257.81,35.56 v260.35,35.56
N$1449  (via drill 0.94)
  Bottom 2.032: v250.19,38.1 v252.73,38.1 v255.27,38.1 v257.81,38.1 v260.35,38.1
N$1450  (via drill 0.94)
  Bottom 2.032: v250.19,40.64 v252.73,40.64 v255.27,40.64 v257.81,40.64 v260.35,40.64
N$1451  (via drill 0.94)
  Bottom 2.032: v250.19,43.18 v252.73,43.18 v255.27,43.18 v257.81,43.18 v260.35,43.18
N$1452  (via drill 0.94)
  Bottom 2.032: v250.19,45.72 v252.73,45.72 v255.27,45.72 v257.81,45.72 v260.35,45.72
N$1453  (via drill 0.94)
  Bottom 2.032: v250.19,48.26 v252.73,48.26 v255.27,48.26 v257.81,48.26 v260.35,48.26
N$1454  (via drill 0.94)
  Bottom 2.032: v250.19,50.8 v252.73,50.8 v255.27,50.8 v257.81,50.8 v260.35,50.8
N$1455  (via drill 0.94)
  Bottom 2.032: v250.19,53.34 v252.73,53.34 v255.27,53.34 v257.81,53.34 v260.35,53.34
N$1456  (via drill 0.94)
  Bottom 2.032: v250.19,55.88 v252.73,55.88 v255.27,55.88 v257.81,55.88 v260.35,55.88
N$1457  (via drill 0.94)
  Bottom 2.032: v250.19,58.42 v252.73,58.42 v255.27,58.42 v257.81,58.42 v260.35,58.42
N$1458  (via drill 0.94)
  Bottom 2.032: v250.19,60.96 v252.73,60.96 v255.27,60.96 v257.81,60.96 v260.35,60.96
N$1459  (via drill 0.94)
  Bottom 2.032: v250.19,63.5 v252.73,63.5 v255.27,63.5 v257.81,63.5 v260.35,63.5
N$1460  (via drill 0.94)
  Bottom 2.032: v250.19,66.04 v252.73,66.04 v255.27,66.04 v257.81,66.04 v260.35,66.04
N$1461  (via drill 0.94)
  Bottom 2.032: v250.19,68.58 v252.73,68.58 v255.27,68.58 v257.81,68.58 v260.35,68.58
N$1462  (via drill 0.94)
  Bottom 2.032: v250.19,71.12 v252.73,71.12 v255.27,71.12 v257.81,71.12 v260.35,71.12
N$1463  (via drill 0.94)
  Bottom 2.032: v250.19,73.66 v252.73,73.66 v255.27,73.66 v257.81,73.66 v260.35,73.66
N$1464  (via drill 0.94)
  Bottom 2.032: v250.19,76.2 v252.73,76.2 v255.27,76.2 v257.81,76.2 v260.35,76.2
N$1465  (via drill 0.94)
  Bottom 2.032: v250.19,78.74 v252.73,78.74 v255.27,78.74 v257.81,78.74 v260.35,78.74
N$1466  (via drill 0.94)
  Bottom 2.032: v250.19,81.28 v252.73,81.28 v255.27,81.28 v257.81,81.28 v260.35,81.28
N$1467  (via drill 0.94)
  Bottom 2.032: v250.19,83.82 v252.73,83.82 v255.27,83.82 v257.81,83.82 v260.35,83.82
N$1468  (via drill 0.94)
  Bottom 2.032: v250.19,86.36 v252.73,86.36 v255.27,86.36 v257.81,86.36 v260.35,86.36
N$1469  (via drill 0.94)
  Bottom 2.032: v250.19,88.9 v252.73,88.9 v255.27,88.9 v257.81,88.9 v260.35,88.9
N$1470  (via drill 0.94)
  Bottom 2.032: v250.19,91.44 v252.73,91.44 v255.27,91.44 v257.81,91.44 v260.35,91.44
N$1471  (via drill 0.94)
  Bottom 2.032: v250.19,93.98 v252.73,93.98 v255.27,93.98 v257.81,93.98 v260.35,93.98
N$1472  (via drill 0.94)
  Bottom 2.032: v250.19,96.52 v252.73,96.52 v255.27,96.52 v257.81,96.52 v260.35,96.52
N$1473  (via drill 0.94)
  Bottom 2.032: v250.19,99.06 v252.73,99.06 v255.27,99.06 v257.81,99.06 v260.35,99.06
N$1474  (via drill 0.94)
  Bottom 2.032: v250.19,101.6 v252.73,101.6 v255.27,101.6 v257.81,101.6 v260.35,101.6
N$1475  (via drill 0.94)
  Bottom 2.032: v250.19,104.14 v252.73,104.14 v255.27,104.14 v257.81,104.14 v260.35,104.14
N$1476  (via drill 0.94)
  Bottom 2.032: v250.19,106.68 v252.73,106.68 v255.27,106.68 v257.81,106.68 v260.35,106.68
N$1477  (via drill 0.94)
  Bottom 2.032: v250.19,109.22 v252.73,109.22 v255.27,109.22 v257.81,109.22 v260.35,109.22
N$1478  (via drill 0.94)
  Bottom 2.032: v250.19,111.76 v252.73,111.76 v255.27,111.76 v257.81,111.76 v260.35,111.76
N$1479  (via drill 0.94)
  Bottom 2.032: v250.19,114.3 v252.73,114.3 v255.27,114.3 v257.81,114.3 v260.35,114.3
N$1480  (via drill 0.94)
  Bottom 2.032: v250.19,116.84 v252.73,116.84 v255.27,116.84 v257.81,116.84 v260.35,116.84
N$1481  (via drill 0.94)
  Bottom 2.032: v250.19,119.38 v252.73,119.38 v255.27,119.38 v257.81,119.38 v260.35,119.38
N$1482  (via drill 0.94)
  Bottom 2.032: v250.19,121.92 v252.73,121.92 v255.27,121.92 v257.81,121.92 v260.35,121.92
N$1483  (via drill 0.94)
  Bottom 2.032: v250.19,124.46 v252.73,124.46 v255.27,124.46 v257.81,124.46 v260.35,124.46
N$1484  (via drill 0.94)
  Bottom 2.032: v250.19,127 v252.73,127 v255.27,127 v257.81,127 v260.35,127
N$1485  (via drill 0.94)
  Bottom 2.032: v250.19,129.54 v252.73,129.54 v255.27,129.54 v257.81,129.54 v260.35,129.54
N$1486  (via drill 0.94)
  Bottom 2.032: v250.19,132.08 v252.73,132.08 v255.27,132.08 v257.81,132.08 v260.35,132.08
N$1487  (via drill 0.94)
  Bottom 2.032: v250.19,134.62 v252.73,134.62 v255.27,134.62 v257.81,134.62 v260.35,134.62
N$1488  (via drill 0.94)
  Bottom 2.032: v250.19,137.16 v252.73,137.16 v255.27,137.16 v257.81,137.16 v260.35,137.16
N$1489  (via drill 0.94)
  Bottom 2.032: v250.19,139.7 v252.73,139.7 v255.27,139.7 v257.81,139.7 v260.35,139.7
N$1490  (via drill 0.94)
  Bottom 2.032: v250.19,142.24 v252.73,142.24 v255.27,142.24 v257.81,142.24 v260.35,142.24
N$1491  (via drill 0.94)
  Bottom 2.032: v250.19,144.78 v252.73,144.78 v255.27,144.78 v257.81,144.78 v260.35,144.78
N$1492  (via drill 0.94)
  Bottom 2.032: v250.19,147.32 v252.73,147.32 v255.27,147.32 v257.81,147.32 v260.35,147.32
N$1493  (via drill 0.94)
  Bottom 2.032: v250.19,149.86 v252.73,149.86 v255.27,149.86 v257.81,149.86 v260.35,149.86
N$1494  (via drill 0.94)
  Bottom 2.032: v250.19,152.4 v252.73,152.4 v255.27,152.4 v257.81,152.4 v260.35,152.4
N$1495  (via drill 0.94)
  Bottom 2.032: v250.19,154.94 v252.73,154.94 v255.27,154.94 v257.81,154.94 v260.35,154.94
N$1496  (via drill 0.94)
  Bottom 2.032: v250.19,157.48 v252.73,157.48 v255.27,157.48 v257.81,157.48 v260.35,157.48
N$1497  (via drill 0.94)
  Bottom 2.032: v250.19,160.02 v252.73,160.02 v255.27,160.02 v257.81,160.02 v260.35,160.02
N$1498  (via drill 0.94)
  Bottom 2.032: v250.19,162.56 v252.73,162.56 v255.27,162.56 v257.81,162.56 v260.35,162.56
N$1499  (via drill 0.94)
  Bottom 2.032: v250.19,165.1 v252.73,165.1 v255.27,165.1 v257.81,165.1 v260.35,165.1
N$1500  (via drill 0.94)
  Bottom 2.032: v250.19,167.64 v252.73,167.64 v255.27,167.64 v257.81,167.64 v260.35,167.64
N$1501  (via drill 0.94)
  Bottom 2.032: v250.19,170.18 v252.73,170.18 v255.27,170.18 v257.81,170.18 v260.35,170.18
N$1502  (via drill 0.94)
  Bottom 2.032: v250.19,172.72 v252.73,172.72 v255.27,172.72 v257.81,172.72 v260.35,172.72
N$1503  (via drill 0.94)
  Bottom 2.032: v250.19,175.26 v252.73,175.26 v255.27,175.26 v257.81,175.26 v260.35,175.26
N$1504  (via drill 0.94)
  Bottom 2.032: v250.19,177.8 v252.73,177.8 v255.27,177.8 v257.81,177.8 v260.35,177.8
N$1505  (via drill 0.94)
  Bottom 2.032: v250.19,180.34 v252.73,180.34 v255.27,180.34 v257.81,180.34 v260.35,180.34
N$1506  (via drill 0.94)
  Bottom 2.032: v250.19,182.88 v252.73,182.88 v255.27,182.88 v257.81,182.88 v260.35,182.88
N$1507  (via drill 0.94)
  Bottom 2.032: v250.19,185.42 v252.73,185.42 v255.27,185.42 v257.81,185.42 v260.35,185.42
N$1508  (via drill 0.94)
  Bottom 2.032: v250.19,187.96 v252.73,187.96 v255.27,187.96 v257.81,187.96 v260.35,187.96
N$1509  (via drill 0.94)
  Bottom 2.032: v250.19,190.5 v252.73,190.5 v255.27,190.5 v257.81,190.5 v260.35,190.5
N$1510  (via drill 0.94)
  Bottom 2.032: v250.19,193.04 v252.73,193.04 v255.27,193.04 v257.81,193.04 v260.35,193.04
N$1511  (via drill 0.94)
  Bottom 2.032: v250.19,195.58 v252.73,195.58 v255.27,195.58 v257.81,195.58 v260.35,195.58
N$1512  (via drill 0.94)
  Bottom 2.032: v250.19,198.12 v252.73,198.12 v255.27,198.12 v257.81,198.12 v260.35,198.12
N$1513  (via drill 0.94)
  Bottom 2.032: v250.19,200.66 v252.73,200.66 v255.27,200.66 v257.81,200.66 v260.35,200.66
N$1514  (via drill 0.94)
  Bottom 2.032: v250.19,203.2 v252.73,203.2 v255.27,203.2 v257.81,203.2 v260.35,203.2
N$1515  (via drill 0.94)
  Bottom 2.032: v250.19,205.74 v252.73,205.74 v255.27,205.74 v257.81,205.74 v260.35,205.74
N$1516  (via drill 0.94)
  Bottom 2.032: v250.19,208.28 v252.73,208.28 v255.27,208.28 v257.81,208.28 v260.35,208.28
N$1517  (via drill 0.94)
  Bottom 2.032: v250.19,210.82 v252.73,210.82 v255.27,210.82 v257.81,210.82 v260.35,210.82
N$1518  (via drill 0.94)
  Bottom 2.032: v250.19,213.36 v252.73,213.36 v255.27,213.36 v257.81,213.36 v260.35,213.36
N$1519  (via drill 0.94)
  Bottom 2.032: v250.19,215.9 v252.73,215.9 v255.27,215.9 v257.81,215.9 v260.35,215.9
N$1520  (via drill 0.94)
  Bottom 2.032: v250.19,218.44 v252.73,218.44 v255.27,218.44 v257.81,218.44 v260.35,218.44
N$1521  (via drill 0.94)
  Bottom 2.032: v250.19,220.98 v252.73,220.98 v255.27,220.98 v257.81,220.98 v260.35,220.98
N$1522  (via drill 0.94)
  Bottom 2.032: v250.19,223.52 v252.73,223.52 v255.27,223.52 v257.81,223.52 v260.35,223.52
N$1523  (via drill 0.94)
  Bottom 2.032: v250.19,226.06 v252.73,226.06 v255.27,226.06 v257.81,226.06 v260.35,226.06
N$1524  (via drill 0.94)
  Bottom 2.032: v250.19,228.6 v252.73,228.6 v255.27,228.6 v257.81,228.6 v260.35,228.6
N$1525  (via drill 0.94)
  Bottom 2.032: v250.19,231.14 v252.73,231.14 v255.27,231.14 v257.81,231.14 v260.35,231.14
N$1526  (via drill 0.94)
  Bottom 2.032: v250.19,233.68 v252.73,233.68 v255.27,233.68 v257.81,233.68 v260.35,233.68
N$1527  (via drill 0.94)
  Bottom 2.032: v250.19,236.22 v252.73,236.22 v255.27,236.22 v257.81,236.22 v260.35,236.22
N$1528  (via drill 0.94)
  Bottom 2.032: v250.19,238.76 v252.73,238.76 v255.27,238.76 v257.81,238.76 v260.35,238.76
N$1529  (via drill 0.94)
  Bottom 2.032: v250.19,241.3 v252.73,241.3 v255.27,241.3 v257.81,241.3 v260.35,241.3
N$1530  (via drill 0.94)
  Bottom 2.032: v250.19,243.84 v252.73,243.84 v255.27,243.84 v257.81,243.84 v260.35,243.84
N$1531  (via drill 0.94)
  Bottom 2.032: v250.19,246.38 v252.73,246.38 v255.27,246.38 v257.81,246.38 v260.35,246.38
N$1532  (via drill 0.94)
  Bottom 2.032: v250.19,248.92 v252.73,248.92 v255.27,248.92 v257.81,248.92 v260.35,248.92
N$1533  (via drill 0.94)
  Bottom 2.032: v250.19,251.46 v252.73,251.46 v255.27,251.46 v257.81,251.46 v260.35,251.46
N$1534  (via drill 0.94)
  Bottom 2.032: v250.19,254 v252.73,254 v255.27,254 v257.81,254 v260.35,254
N$1535  (via drill 0.94)
  Bottom 2.032: v250.19,256.54 v252.73,256.54 v255.27,256.54 v257.81,256.54 v260.35,256.54
N$1536  (via drill 0.94)
  Bottom 2.032: v250.19,259.08 v252.73,259.08 v255.27,259.08 v257.81,259.08 v260.35,259.08
N$1537  (via drill 0.94)
  Bottom 2.032: v250.19,261.62 v252.73,261.62 v255.27,261.62 v257.81,261.62 v260.35,261.62
N$1538  (via drill 0.94)
  Bottom 2.032: v250.19,264.16 v252.73,264.16 v255.27,264.16 v257.81,264.16 v260.35,264.16
N$1539  (via drill 0.94)
  Bottom 2.032: v250.19,266.7 v252.73,266.7 v255.27,266.7 v257.81,266.7 v260.35,266.7
N$1540  (via drill 0.94)
  Bottom 2.032: v250.19,269.24 v252.73,269.24 v255.27,269.24 v257.81,269.24 v260.35,269.24
N$1541  (via drill 0.94)
  Bottom 2.032: v250.19,271.78 v252.73,271.78 v255.27,271.78 v257.81,271.78 v260.35,271.78
N$1542  (via drill 0.94)
  Bottom 2.032: v250.19,274.32 v252.73,274.32 v255.27,274.32 v257.81,274.32 v260.35,274.32
N$1543  (via drill 0.94)
  Bottom 2.032: v250.19,276.86 v252.73,276.86 v255.27,276.86 v257.81,276.86 v260.35,276.86
N$1544  (via drill 0.94)
  Bottom 2.032: v262.89,12.7 v265.43,12.7 v267.97,12.7 v270.51,12.7 v273.05,12.7
N$1545  (via drill 0.94)
  Bottom 2.032: v262.89,15.24 v265.43,15.24 v267.97,15.24 v270.51,15.24 v273.05,15.24
N$1546  (via drill 0.94)
  Bottom 2.032: v262.89,17.78 v265.43,17.78 v267.97,17.78 v270.51,17.78 v273.05,17.78
N$1547  (via drill 0.94)
  Bottom 2.032: v262.89,20.32 v265.43,20.32 v267.97,20.32 v270.51,20.32 v273.05,20.32
N$1548  (via drill 0.94)
  Bottom 2.032: v262.89,22.86 v265.43,22.86 v267.97,22.86 v270.51,22.86 v273.05,22.86
N$1549  (via drill 0.94)
  Bottom 2.032: v262.89,25.4 v265.43,25.4 v267.97,25.4 v270.51,25.4 v273.05,25.4
N$1550  (via drill 0.94)
  Bottom 2.032: v262.89,27.94 v265.43,27.94 v267.97,27.94 v270.51,27.94 v273.05,27.94
N$1551  (via drill 0.94)
  Bottom 2.032: v262.89,30.48 v265.43,30.48 v267.97,30.48 v270.51,30.48 v273.05,30.48
N$1552  (via drill 0.94)
  Bottom 2.032: v262.89,33.02 v265.43,33.02 v267.97,33.02 v270.51,33.02 v273.05,33.02
N$1553  (via drill 0.94)
  Bottom 2.032: v262.89,35.56 v265.43,35.56 v267.97,35.56 v270.51,35.56 v273.05,35.56
N$1554  (via drill 0.94)
  Bottom 2.032: v262.89,38.1 v265.43,38.1 v267.97,38.1 v270.51,38.1 v273.05,38.1
N$1555  (via drill 0.94)
  Bottom 2.032: v262.89,40.64 v265.43,40.64 v267.97,40.64 v270.51,40.64 v273.05,40.64
N$1556  (via drill 0.94)
  Bottom 2.032: v262.89,43.18 v265.43,43.18 v267.97,43.18 v270.51,43.18 v273.05,43.18
N$1557  (via drill 0.94)
  Bottom 2.032: v262.89,45.72 v265.43,45.72 v267.97,45.72 v270.51,45.72 v273.05,45.72
N$1558  (via drill 0.94)
  Bottom 2.032: v262.89,48.26 v265.43,48.26 v267.97,48.26 v270.51,48.26 v273.05,48.26
N$1559  (via drill 0.94)
  Bottom 2.032: v262.89,50.8 v265.43,50.8 v267.97,50.8 v270.51,50.8 v273.05,50.8
N$1560  (via drill 0.94)
  Bottom 2.032: v262.89,53.34 v265.43,53.34 v267.97,53.34 v270.51,53.34 v273.05,53.34
N$1561  (via drill 0.94)
  Bottom 2.032: v262.89,55.88 v265.43,55.88 v267.97,55.88 v270.51,55.88 v273.05,55.88
N$1562  (via drill 0.94)
  Bottom 2.032: v262.89,58.42 v265.43,58.42 v267.97,58.42 v270.51,58.42 v273.05,58.42
N$1563  (via drill 0.94)
  Bottom 2.032: v262.89,60.96 v265.43,60.96 v267.97,60.96 v270.51,60.96 v273.05,60.96
N$1564  (via drill 0.94)
  Bottom 2.032: v262.89,63.5 v265.43,63.5 v267.97,63.5 v270.51,63.5 v273.05,63.5
N$1565  (via drill 0.94)
  Bottom 2.032: v262.89,66.04 v265.43,66.04 v267.97,66.04 v270.51,66.04 v273.05,66.04
N$1566  (via drill 0.94)
  Bottom 2.032: v262.89,68.58 v265.43,68.58 v267.97,68.58 v270.51,68.58 v273.05,68.58
N$1567  (via drill 0.94)
  Bottom 2.032: v262.89,71.12 v265.43,71.12 v267.97,71.12 v270.51,71.12 v273.05,71.12
N$1568  (via drill 0.94)
  Bottom 2.032: v262.89,73.66 v265.43,73.66 v267.97,73.66 v270.51,73.66 v273.05,73.66
N$1569  (via drill 0.94)
  Bottom 2.032: v262.89,76.2 v265.43,76.2 v267.97,76.2 v270.51,76.2 v273.05,76.2
N$1570  (via drill 0.94)
  Bottom 2.032: v262.89,78.74 v265.43,78.74 v267.97,78.74 v270.51,78.74 v273.05,78.74
N$1571  (via drill 0.94)
  Bottom 2.032: v262.89,81.28 v265.43,81.28 v267.97,81.28 v270.51,81.28 v273.05,81.28
N$1572  (via drill 0.94)
  Bottom 2.032: v262.89,83.82 v265.43,83.82 v267.97,83.82 v270.51,83.82 v273.05,83.82
N$1573  (via drill 0.94)
  Bottom 2.032: v262.89,86.36 v265.43,86.36 v267.97,86.36 v270.51,86.36 v273.05,86.36
N$1574  (via drill 0.94)
  Bottom 2.032: v262.89,88.9 v265.43,88.9 v267.97,88.9 v270.51,88.9 v273.05,88.9
N$1575  (via drill 0.94)
  Bottom 2.032: v262.89,91.44 v265.43,91.44 v267.97,91.44 v270.51,91.44 v273.05,91.44
N$1576  (via drill 0.94)
  Bottom 2.032: v262.89,93.98 v265.43,93.98 v267.97,93.98 v270.51,93.98 v273.05,93.98
N$1577  (via drill 0.94)
  Bottom 2.032: v262.89,96.52 v265.43,96.52 v267.97,96.52 v270.51,96.52 v273.05,96.52
N$1578  (via drill 0.94)
  Bottom 2.032: v262.89,99.06 v265.43,99.06 v267.97,99.06 v270.51,99.06 v273.05,99.06
N$1579  (via drill 0.94)
  Bottom 2.032: v262.89,101.6 v265.43,101.6 v267.97,101.6 v270.51,101.6 v273.05,101.6
N$1580  (via drill 0.94)
  Bottom 2.032: v262.89,104.14 v265.43,104.14 v267.97,104.14 v270.51,104.14 v273.05,104.14
N$1581  (via drill 0.94)
  Bottom 2.032: v262.89,106.68 v265.43,106.68 v267.97,106.68 v270.51,106.68 v273.05,106.68
N$1582  (via drill 0.94)
  Bottom 2.032: v262.89,109.22 v265.43,109.22 v267.97,109.22 v270.51,109.22 v273.05,109.22
N$1583  (via drill 0.94)
  Bottom 2.032: v262.89,111.76 v265.43,111.76 v267.97,111.76 v270.51,111.76 v273.05,111.76
N$1584  (via drill 0.94)
  Bottom 2.032: v262.89,114.3 v265.43,114.3 v267.97,114.3 v270.51,114.3 v273.05,114.3
N$1585  (via drill 0.94)
  Bottom 2.032: v262.89,116.84 v265.43,116.84 v267.97,116.84 v270.51,116.84 v273.05,116.84
N$1586  (via drill 0.94)
  Bottom 2.032: v262.89,119.38 v265.43,119.38 v267.97,119.38 v270.51,119.38 v273.05,119.38
N$1587  (via drill 0.94)
  Bottom 2.032: v262.89,121.92 v265.43,121.92 v267.97,121.92 v270.51,121.92 v273.05,121.92
N$1588  (via drill 0.94)
  Bottom 2.032: v262.89,124.46 v265.43,124.46 v267.97,124.46 v270.51,124.46 v273.05,124.46
N$1589  (via drill 0.94)
  Bottom 2.032: v262.89,127 v265.43,127 v267.97,127 v270.51,127 v273.05,127
N$1590  (via drill 0.94)
  Bottom 2.032: v262.89,129.54 v265.43,129.54 v267.97,129.54 v270.51,129.54 v273.05,129.54
N$1591  (via drill 0.94)
  Bottom 2.032: v262.89,132.08 v265.43,132.08 v267.97,132.08 v270.51,132.08 v273.05,132.08
N$1592  (via drill 0.94)
  Bottom 2.032: v262.89,134.62 v265.43,134.62 v267.97,134.62 v270.51,134.62 v273.05,134.62
N$1593  (via drill 0.94)
  Bottom 2.032: v262.89,137.16 v265.43,137.16 v267.97,137.16 v270.51,137.16 v273.05,137.16
N$1594  (via drill 0.94)
  Bottom 2.032: v262.89,139.7 v265.43,139.7 v267.97,139.7 v270.51,139.7 v273.05,139.7
N$1595  (via drill 0.94)
  Bottom 2.032: v262.89,142.24 v265.43,142.24 v267.97,142.24 v270.51,142.24 v273.05,142.24
N$1596  (via drill 0.94)
  Bottom 2.032: v262.89,144.78 v265.43,144.78 v267.97,144.78 v270.51,144.78 v273.05,144.78
N$1597  (via drill 0.94)
  Bottom 2.032: v262.89,147.32 v265.43,147.32 v267.97,147.32 v270.51,147.32 v273.05,147.32
N$1598  (via drill 0.94)
  Bottom 2.032: v262.89,149.86 v265.43,149.86 v267.97,149.86 v270.51,149.86 v273.05,149.86
N$1599  (via drill 0.94)
  Bottom 2.032: v262.89,152.4 v265.43,152.4 v267.97,152.4 v270.51,152.4 v273.05,152.4
N$1600  (via drill 0.94)
  Bottom 2.032: v262.89,154.94 v265.43,154.94 v267.97,154.94 v270.51,154.94 v273.05,154.94
N$1601  (via drill 0.94)
  Bottom 2.032: v262.89,157.48 v265.43,157.48 v267.97,157.48 v270.51,157.48 v273.05,157.48
N$1602  (via drill 0.94)
  Bottom 2.032: v262.89,160.02 v265.43,160.02 v267.97,160.02 v270.51,160.02 v273.05,160.02
N$1603  (via drill 0.94)
  Bottom 2.032: v262.89,162.56 v265.43,162.56 v267.97,162.56 v270.51,162.56 v273.05,162.56
N$1604  (via drill 0.94)
  Bottom 2.032: v262.89,165.1 v265.43,165.1 v267.97,165.1 v270.51,165.1 v273.05,165.1
N$1605  (via drill 0.94)
  Bottom 2.032: v262.89,167.64 v265.43,167.64 v267.97,167.64 v270.51,167.64 v273.05,167.64
N$1606  (via drill 0.94)
  Bottom 2.032: v262.89,170.18 v265.43,170.18 v267.97,170.18 v270.51,170.18 v273.05,170.18
N$1607  (via drill 0.94)
  Bottom 2.032: v262.89,172.72 v265.43,172.72 v267.97,172.72 v270.51,172.72 v273.05,172.72
N$1608  (via drill 0.94)
  Bottom 2.032: v262.89,175.26 v265.43,175.26 v267.97,175.26 v270.51,175.26 v273.05,175.26
N$1609  (via drill 0.94)
  Bottom 2.032: v262.89,177.8 v265.43,177.8 v267.97,177.8 v270.51,177.8 v273.05,177.8
N$1610  (via drill 0.94)
  Bottom 2.032: v262.89,180.34 v265.43,180.34 v267.97,180.34 v270.51,180.34 v273.05,180.34
N$1611  (via drill 0.94)
  Bottom 2.032: v262.89,182.88 v265.43,182.88 v267.97,182.88 v270.51,182.88 v273.05,182.88
N$1612  (via drill 0.94)
  Bottom 2.032: v262.89,185.42 v265.43,185.42 v267.97,185.42 v270.51,185.42 v273.05,185.42
N$1613  (via drill 0.94)
  Bottom 2.032: v262.89,187.96 v265.43,187.96 v267.97,187.96 v270.51,187.96 v273.05,187.96
N$1614  (via drill 0.94)
  Bottom 2.032: v262.89,190.5 v265.43,190.5 v267.97,190.5 v270.51,190.5 v273.05,190.5
N$1615  (via drill 0.94)
  Bottom 2.032: v262.89,193.04 v265.43,193.04 v267.97,193.04 v270.51,193.04 v273.05,193.04
N$1616  (via drill 0.94)
  Bottom 2.032: v262.89,195.58 v265.43,195.58 v267.97,195.58 v270.51,195.58 v273.05,195.58
N$1617  (via drill 0.94)
  Bottom 2.032: v262.89,198.12 v265.43,198.12 v267.97,198.12 v270.51,198.12 v273.05,198.12
N$1618  (via drill 0.94)
  Bottom 2.032: v262.89,200.66 v265.43,200.66 v267.97,200.66 v270.51,200.66 v273.05,200.66
N$1619  (via drill 0.94)
  Bottom 2.032: v262.89,203.2 v265.43,203.2 v267.97,203.2 v270.51,203.2 v273.05,203.2
N$1620  (via drill 0.94)
  Bottom 2.032: v262.89,205.74 v265.43,205.74 v267.97,205.74 v270.51,205.74 v273.05,205.74
N$1621  (via drill 0.94)
  Bottom 2.032: v262.89,208.28 v265.43,208.28 v267.97,208.28 v270.51,208.28 v273.05,208.28
N$1622  (via drill 0.94)
  Bottom 2.032: v262.89,210.82 v265.43,210.82 v267.97,210.82 v270.51,210.82 v273.05,210.82
N$1623  (via drill 0.94)
  Bottom 2.032: v262.89,213.36 v265.43,213.36 v267.97,213.36 v270.51,213.36 v273.05,213.36
N$1624  (via drill 0.94)
  Bottom 2.032: v262.89,215.9 v265.43,215.9 v267.97,215.9 v270.51,215.9 v273.05,215.9
N$1625  (via drill 0.94)
  Bottom 2.032: v262.89,218.44 v265.43,218.44 v267.97,218.44 v270.51,218.44 v273.05,218.44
